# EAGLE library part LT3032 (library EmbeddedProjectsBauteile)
LINEAR TECHNOLOGY - LT3032IDE#PBF - LDO-REGLER
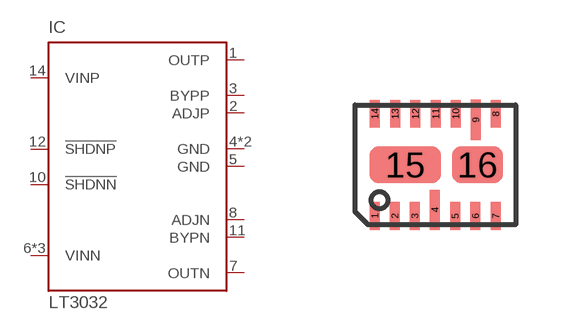
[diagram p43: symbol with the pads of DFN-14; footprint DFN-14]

Designator prefix IC

## LT3032 (EP: 401425)  [DFN-14]
1  OUTP  out
2  ADJP  in
3  BYPP  in
4  GND  pwr
5  GND  pwr
6  VINN  in
7  OUTN  out
8  ADJN  in
9  VINN  in
10  !SHDNN  in
11  BYPN  in
12  !SHDNP  in
14  VINP  in
15  GND  pwr
16  VINN  in

## Footprint DFN-14 (pad centres in mm)
smd 0.25 x 0.7: 1 -1.512,-1.277; 2 -1.012,-1.277; 3 -0.512,-1.277; 5 0.496,-1.277; 6 1.004,-1.277; 7 1.512,-1.277; 8 1.512,1.277; 10 0.512,1.277; 11 0.012,1.277; 12 -0.496,1.277; 13 -1.004,1.277; 14 -1.512,1.277
smd 0.25 x 1: 4 -0.012,-1.127; 9 1.012,1.127
smd 1.778 x 0.914: 15 -0.75,0
smd 1.27 x 0.914: 16 1.05,0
